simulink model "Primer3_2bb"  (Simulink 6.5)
settings: Solver=ode23t  SolverMode=SingleTasking  StartTime=0.0  StopTime=0.6  RelTol=1e-3  AbsTol=1e-6
undefined symbols (not defined in the file or in its folder): blocks, Continuous, powergui, ZData
libraries: powerlib x13

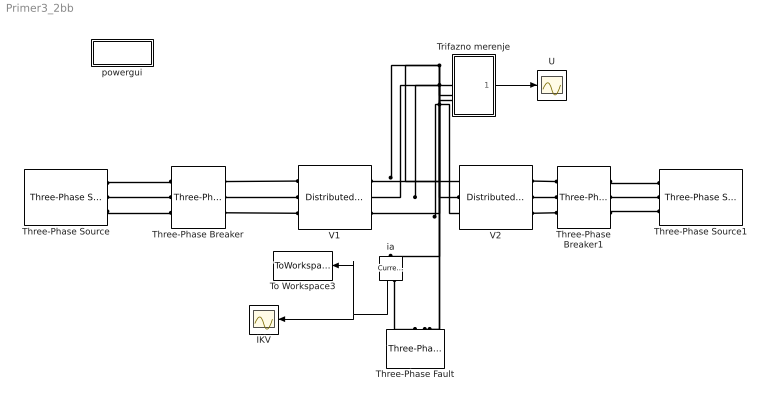
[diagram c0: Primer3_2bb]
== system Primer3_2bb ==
  IKV : Scope
  Three-Phase Breaker : powerlib/Elements/Three-Phase Breaker  DialogController=PMDialogs.PMDefaultMaskDlg  SystemSampleTime=-1  InitialState=closed  SwitchA=on  SwitchB=off  SwitchC=off  SwitchTimes="[ 10/50  20/50 ]"  External=off  BreakerResistance=0.001  SnubberResistance=1e6  SnubberCapacitance=inf  Measurements=None
  Three-Phase Breaker1 : powerlib/Elements/Three-Phase Breaker  Orientation=left  DialogController=PMDialogs.PMDefaultMaskDlg  SystemSampleTime=-1  InitialState=closed  SwitchA=on  SwitchB=off  SwitchC=off  SwitchTimes="[ 10/50  20/50 ]"  External=off  BreakerResistance=0.001  SnubberResistance=1e6  SnubberCapacitance=inf  Measurements=None
  Three-Phase Fault : powerlib/Elements/Three-Phase Fault  Orientation=down  DialogController=PMDialogs.PMDefaultMaskDlg  SystemSampleTime=-1  FaultA=on  FaultB=off  FaultC=off  FaultResistance=0.001  GroundFault=on  GroundResistance=0.001  External=off  SwitchStatus=[1 0]  SwitchTimes=[ 3/50 15/50]  InitialStates=[0 0 1]  SnubberResistance=1e6  SnubberCapacitance=inf  Measurements=None
  Three-Phase Source : powerlib/Electrical Sources/Three-Phase Source  DialogController=PMDialogs.PMDefaultMaskDlg  SystemSampleTime=-1  Voltage=410e3  PhaseAngle=0  Frequency=50  InternalConnection=Yg  SpecifyImpedance=on  Resistance=0.8929  Inductance=16.58e-3  ShortCircuitLevel=sqrt(3)*400e3*16e3  BaseVoltage=400e3  XRratio=10
  Three-Phase Source1 : powerlib/Electrical Sources/Three-Phase Source  Orientation=left  DialogController=PMDialogs.PMDefaultMaskDlg  SystemSampleTime=-1  Voltage=395e3  PhaseAngle=-2.5  Frequency=50  InternalConnection=Yg  SpecifyImpedance=on  Resistance=0.8929  Inductance=16.58e-3  ShortCircuitLevel=sqrt(3)*400e3*14e3  BaseVoltage=400e3  XRratio=10
  To Workspace3 : ToWorkspace  VariableName=ikv  SampleTime=-1  SaveFormat=Array
  Trifazno merenje : Subsystem
  U : Scope
  V1 : powerlib/Elements/Distributed Parameters Line  DialogController=PMDialogs.PMDefaultMaskDlg  SystemSampleTime=-1  Phases=3  Frequency=50  Resistance=[0.029983 0.29405]  Inductance=[0.0010055 0.0025377]  Capacitance=[1.1784e-008 8.6541e-009]  Length=113.5/2  x1=[0 5.07182191408931e-011 178450.018618737 -366847.020662789;5.31896283741607e-005 5.22461244981202e-011 184554.839172681 -363814.04185674;0.000106379256748321 5.37594417922576e-011 190608.12867694 -360679.479588827;0.000159568885122482 5.52577484777409e-011 196608.19694358 -357444.209085539;0.000212758513496643 5.67406262002393e-011 202553.368645001 -354109.133692926;0.000265948141870804 5.8207660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  x2=[0 7.95772463746972e-011 172736.109706228 -365994.140775089;5.31896283741607e-005 8.69975667901571e-011 178827.47700141 -363056.756096686;0.000106379256748321 9.43935959111874e-011 184868.912430032 -360017.999404301;0.000159568885122482 1.01763268632664e-010 190858.729114034 -356878.719173774;0.000212758513496643 1.09104527208645e-010 196795.254588242 -353639.791948936;0.000265948141870804 1.16415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  x3=[0 -7.35569200775802e-012 586.956046574638 -949.442634179255;5.31896283741607e-005 -7.27673326092948e-012 602.738564141194 -939.502495741647;0.000106379256748321 -7.19574271853874e-012 618.352786197131 -929.300031211674;0.000159568885122482 -7.11274299461036e-012 633.79435296919 -918.838089301994;0.000212758513496643 -7.0277572641687e-012 649.058952892591 -908.119591176045;0.000265948141870804 -6.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  x4=[0 6.50938879444972e-012 533.264836498686 -1585.21009257673;5.31896283741607e-005 6.44250381180511e-012 559.678038947736 -1576.07833440242;0.000106379256748321 6.37381996555167e-012 585.934969163764 -1566.50650664597;0.000159568885122482 6.30335643346176e-012 612.028295736867 -1556.49728193483;0.000212758513496643 6.23113289022821e-012 637.950732938237 -1546.05345502562;0.000265948141870804 6.1571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  x5=0.000265948141870804  Measurements=None
  V2 : powerlib/Elements/Distributed Parameters Line  DialogController=PMDialogs.PMDefaultMaskDlg  SystemSampleTime=-1  Phases=3  Frequency=50  Resistance=[0.029983 0.29405]  Inductance=[0.0010055 0.0025377]  Capacitance=[1.1784e-008 8.6541e-009]  Length=113.5/2  x1=[0 7.95772463746972e-011 172736.109706228 -365994.140775089;5.31896283741607e-005 8.69975667901571e-011 178827.47700141 -363056.756096686;0.000106379256748321 9.43935959111874e-011 184868.912430032 -360017.999404301;0.000159568885122482 1.01763268632664e-010 190858.729114034 -356878.719173774;0.000212758513496643 1.09104527208645e-010 196795.254588242 -353639.791948936;0.000265948141870804 1.16415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  x2=[0 -4.96471005783232e-011 166509.443707765 -363699.090775954;5.31896283741607e-005 -4.55615980335971e-011 172563.331767605 -360866.069344832;0.000106379256748321 -4.1463373866493e-011 178569.037023553 -357932.287579098;0.000159568885122482 -3.73535723753349e-011 184524.882574059 -354898.564643695;0.000212758513496643 -3.32333410910454e-011 190429.205439304 -351765.747608946;0.000265948141870804 -2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  x3=[0 1.20076442730669e-012 644.436346866559 -910.109116757232;5.31896283741607e-005 1.14033199404794e-012 659.553606600823 -899.214017677211;0.000106379256748321 1.07958115946791e-012 674.486707036831 -888.067841776716;0.000159568885122482 1.01852888629858e-012 689.231478582803 -876.673701269694;0.000212758513496643 9.57192221439062e-013 703.783804231792 -865.034777606293;0.000265948141870804 8.9558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  x4=[0 -3.65792780299756e-012 435.41541414618 -1612.56297375388;5.31896283741607e-005 -3.57759592315401e-012 462.299323032339 -1605.06238605291;0.000106379256748321 -3.49626511381019e-012 489.054149584536 -1597.11363589827;0.000159568885122482 -3.41395808399932e-012 515.672423371203 -1588.71894272477;0.000212758513496643 -3.33069781533307e-012 542.146712088775 -1579.88065048261;0.000265948141870804 -3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  x5=0.000265948141870804  Measurements=None
  ia : powerlib/Measurements/Current Measurement  Orientation=down  DialogController=PMDialogs.PMDefaultMaskDlg  SystemSampleTime=-1  PhasorSimulation=off  OutputType=Complex  PSBequivalent=0
  powergui : Subsystem  AncestorBlock=powerlib/powergui  InitFcn=powergui( 'InitFcn_Callback' , gcb , 0 , [ ] );  mask(PSB option menu block){SimulationMode=Continuous, SampleTime=50e-6, echomessages=off, RestoreLinks=warning, x0status=blocks, Frange=[0:2:500], Ylog=off, Xlog=on, ShowGrid=off, save=off, variable=ZData, structure=, ZoomFFT=on, StartTime=0.0, cycles=1, DisplayStyle=1, fundamental=60, FreqAxis=off, MaxFrequency=1000, frequencyindice=50, frequencyindicesteady=1, RmsSteady=1, display=off, Ts=0, frequency=60, methode=off, HookPort=off, Interpol=off}
      mask prompts: SimulationMode "Simulation mode"; SampleTime "Sample time Ts (when simulation mode is Discrete) (s)"; echomessages "Echo  Messages"; RestoreLinks "Restore disabled links"; x0status "Initial electrical states status"; Frange "Impedance tool: Frequency Range"; Ylog "Impedance tool: Log impedance"; Xlog "Impedance tool: log Frequency"; ShowGrid "Impedance tool: grid"; save "Impedance tool: Save Data To Workspace"; variable "Impedance tool: Variable Name"; structure "Structure Name (PSBFFTSCOPE)"; ZoomFFT "ZoomFFT (PSBFFTSCOPE)"; StartTime "Start Time (PSBFFTSCOPE)"; cycles "Cycles (PSBFFTSCOPE)"; DisplayStyle "Display style (PSBFFTSCOPE)"; fundamental "Fundamental (PSBFFTSCOPE)"; FreqAxis "Frequency Axis (PSBFFTSCOPE)"; MaxFrequency "Max Frequency (PSBFFTSCOPE)"; frequencyindice "Load flow frequency (Hz)"; frequencyindicesteady "Frequency indice (STEADYSTATE)"; RmsSteady "RMS display (STEADYSTATE)"; display "Display Results"; Ts "OBSOLETE 1"; frequency "Phasor frequency (Hz)"; methode "Phasor simulation"; HookPort "Hook port"; Interpol "Interpolate"
      mask init:
      | powerlibroot = which('powersysdomain');
      | PSBroot = powerlibroot(1:end-16);
      | %
      | switch SimulationMode
      | 	case 1
      | 		message=sprintf('Continuous');
      | 	case 2
      |         SampleTimeeval=evalin('base',SampleTime,'NaN');
      |         if isnan(SampleTimeeval)
      |             message=sprintf('Warning !!,\nUndefined sample time');
      |         else
      |             message=sprintf('Discrete,\nTs = %.4g s.',SampleTimeeval);
      |         end
      | 	case 3
      | 		message=sprintf('Phasors');
      | end
      | if strcmp(bdroot,'powerlib')
      |   message='powergui';
      | end
      | power_initmask();
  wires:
  ia/1 -> IKV/1, To Workspace3/1
  Trifazno merenje/1(Izlez) -> U/1
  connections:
  Three-Phase Breaker/RConn1 -- V1/LConn1
  Three-Phase Source/RConn1 -- Three-Phase Breaker/LConn1
  Three-Phase Source/RConn2 -- Three-Phase Breaker/LConn2
  Three-Phase Source/RConn3 -- Three-Phase Breaker/LConn3
  V1/LConn2 -- Three-Phase Breaker/RConn2
  V1/LConn3 -- Three-Phase Breaker/RConn3
  Three-Phase Breaker1/LConn1 -- Three-Phase Source1/RConn1
  Three-Phase Breaker1/LConn2 -- Three-Phase Source1/RConn2
  Three-Phase Breaker1/LConn3 -- Three-Phase Source1/RConn3
  Trifazno merenje/LConn1 -- V2/LConn1 -- V1/RConn1 -- ia/LConn1
  Trifazno merenje/LConn2 -- V1/RConn2 -- V2/LConn2 -- Three-Phase Fault/LConn2
  Trifazno merenje/LConn3 -- V2/LConn3 -- V1/RConn3 -- Three-Phase Fault/LConn3
  Three-Phase Breaker1/RConn1 -- V2/RConn1
  V2/RConn2 -- Three-Phase Breaker1/RConn2
  V2/RConn3 -- Three-Phase Breaker1/RConn3
  ia/RConn1 -- Three-Phase Fault/LConn1

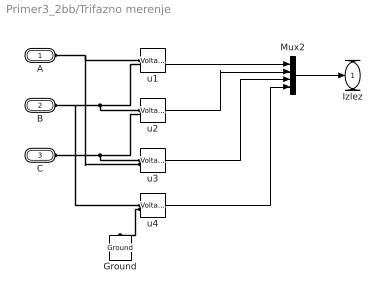
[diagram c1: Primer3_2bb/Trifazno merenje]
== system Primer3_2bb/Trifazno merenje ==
  Ground : powerlib/Elements/Ground  Orientation=down  DialogController=PMDialogs.PMDefaultMaskDlg  PhysicalDomain=powersysdomain  SubClassName=unknown  LeftPortType=p1  RightPortType=p1  LConnTagsString=a
  Mux2 : Mux
  u{1..4} (4 alike) : powerlib/Measurements/Voltage Measurement  Tag=PoWeRsYsTeMmEaSuReMeNt  DialogController=PMDialogs.PMDefaultMaskDlg  SystemSampleTime=-1  PhasorSimulation=off  OutputType=Magnitude  PSBequivalent=0
  A : PMIOPort  Port=1  Side=Left
  B : PMIOPort  Port=2  Side=Left
  C : PMIOPort  Port=3  Side=Left
  Izlez : Outport
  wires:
  u1/1 -> Mux2/1
  u2/1 -> Mux2/2
  Mux2/1 -> Izlez/1
  u3/1 -> Mux2/3
  u4/1 -> Mux2/4
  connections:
  A/RConn1 -- u1/LConn1 -- u3/LConn2
  B/RConn1 -- u2/LConn1 -- u1/LConn2 -- u4/LConn1
  C/RConn1 -- u3/LConn1 -- u2/LConn2
  u4/LConn2 -- Ground/LConn1

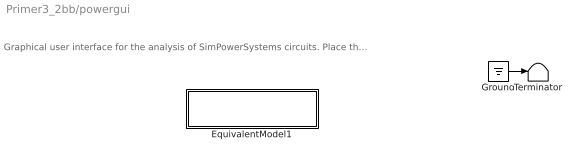
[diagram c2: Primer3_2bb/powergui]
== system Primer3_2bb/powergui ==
  note: Graphical user interface for the analysis of SimPowerSystems circuits. Place the Powergui block in the top-level of your model and double-click on it to open the GUI.
  EquivalentModel1 : Subsystem
  Ground : Ground
  Terminator : Terminator
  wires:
  Ground/1 -> Terminator/1

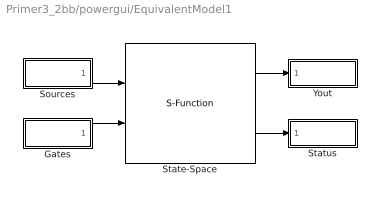
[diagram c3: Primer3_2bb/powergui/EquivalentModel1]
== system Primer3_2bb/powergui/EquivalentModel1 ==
  Gates : Subsystem
  Sources : Subsystem
  State-Space : S-Function  FunctionName=sfun_spssw_contc  Parameters=A, B, C, D, x0, SwitchResistance ,SwitchType, SwitchGateInitialValue, OutputsToResetToZero
  Status : Subsystem
  Yout : Subsystem
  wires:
  Gates/1(gates) -> State-Space/2
  Sources/1(u) -> State-Space/1
  State-Space/2 -> Status/1(status)
  State-Space/1 -> Yout/1(v,i)

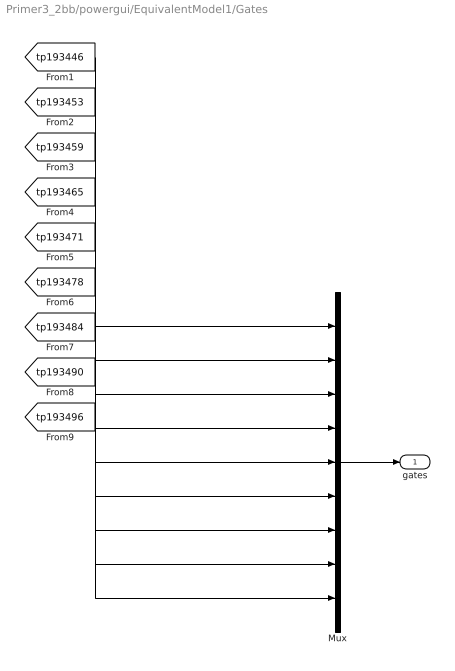
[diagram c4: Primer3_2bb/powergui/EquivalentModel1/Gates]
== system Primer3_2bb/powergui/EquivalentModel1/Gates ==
  Mux : Mux  Inputs=[1 1 1 1 1 1 1 1 1]
  gates : Outport
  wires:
  Mux/1 -> gates/1
  [tp193446] -> Mux/1
  [tp193453] -> Mux/2
  [tp193459] -> Mux/3
  [tp193465] -> Mux/4
  [tp193471] -> Mux/5
  [tp193478] -> Mux/6
  [tp193484] -> Mux/7
  [tp193490] -> Mux/8
  [tp193496] -> Mux/9

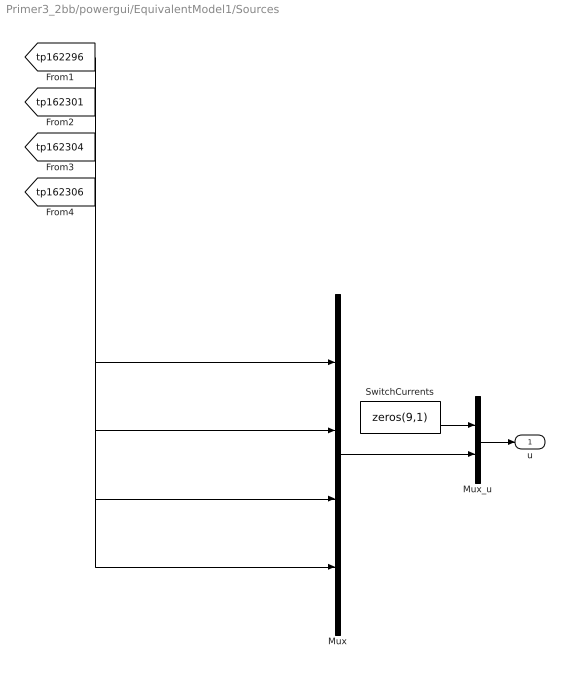
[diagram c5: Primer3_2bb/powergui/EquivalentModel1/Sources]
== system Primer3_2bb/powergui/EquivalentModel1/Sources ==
  Mux : Mux  Inputs=[6 6 3 3]
  Mux_u : Mux  Inputs=[9 18]
  SwitchCurrents : Constant  Value=zeros(9,1)  OutDataType=sfix(16)  ConRadixGroup=Use specified scaling  OutScaling=2^0  SampleTime=inf  FramePeriod=inf
  u : Outport
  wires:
  Mux/1 -> Mux_u/2
  SwitchCurrents/1 -> Mux_u/1
  Mux_u/1 -> u/1
  [tp162296] -> Mux/1
  [tp162301] -> Mux/2
  [tp162304] -> Mux/3
  [tp162306] -> Mux/4

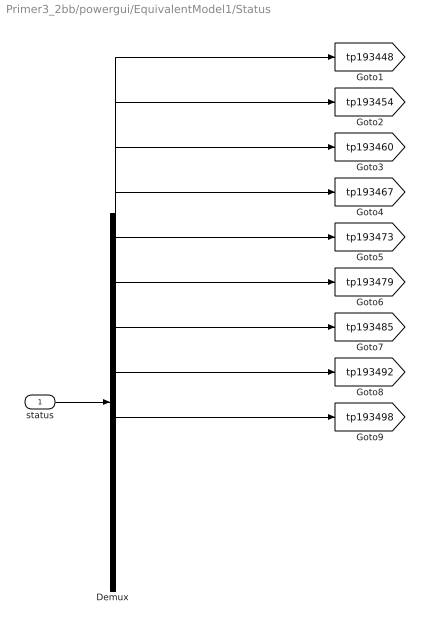
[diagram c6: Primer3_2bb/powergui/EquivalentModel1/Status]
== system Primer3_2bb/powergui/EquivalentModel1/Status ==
  status : Inport
  Demux : Demux  Outputs=[1 1 1 1 1 1 1 1 1]
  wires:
  status/1 -> Demux/1
  Demux/1 -> [tp193448]
  Demux/2 -> [tp193454]
  Demux/3 -> [tp193460]
  Demux/4 -> [tp193467]
  Demux/5 -> [tp193473]
  Demux/6 -> [tp193479]
  Demux/7 -> [tp193485]
  Demux/8 -> [tp193492]
  Demux/9 -> [tp193498]

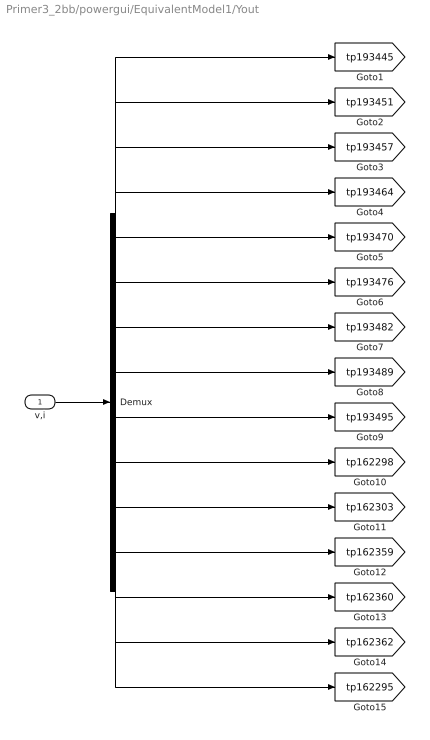
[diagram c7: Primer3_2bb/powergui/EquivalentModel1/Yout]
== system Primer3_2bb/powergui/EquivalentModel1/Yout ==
  v,i : Inport
  Demux : Demux  Outputs=[1 1 1 1 1 1 1 1 1 6 6 1 1 1 1]
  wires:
  v,i/1 -> Demux/1
  Demux/1 -> [tp193445]
  Demux/2 -> [tp193451]
  Demux/3 -> [tp193457]
  Demux/4 -> [tp193464]
  Demux/5 -> [tp193470]
  Demux/6 -> [tp193476]
  Demux/7 -> [tp193482]
  Demux/8 -> [tp193489]
  Demux/9 -> [tp193495]
  Demux/10 -> [tp162298]
  Demux/11 -> [tp162303]
  Demux/12 -> [tp162359]
  Demux/13 -> [tp162360]
  Demux/14 -> [tp162362]
  Demux/15 -> [tp162295]
